TYPE ST_States :
STRUCT
	ManualModeIsActive:				BOOL;(*手动模式*)
	AutoModeIsActive:				BOOL;(*自动模式*)
	MachineRunInCycle:				BOOL;(*自动运行中*)
	GoPauseState:					BOOL;(*请求暂停记忆*)
	AutoStoping:					BOOL;(*自动停机中*)
	ResetAlarm:						BOOL;(*报警复位*)
	GoHome:							BOOL;(*请求找原点*)


	(*电机*)
	HomeDone:						BOOL;(*原点完成*)
	Motor_PowerOn:				BOOL;(*上电完成*)
	Motor_HomeDone:				BOOL;(*原点完成*)
	Motor_SwError:				BOOL;(*电机NC软件出错*)
	Motor_SwErrId:				UDINT;
	Motor_Limit:				BOOL;(*电机限位*)
	Motor_HwError:				BOOL;(*电机硬件出错*)

	Hmi_btHome:						BOOL;(*画面按钮*)(*回原点*)
	Hmi_btAutoRun:					BOOL;(*画面按钮*)(*开始*)
	Hmi_btAutoStop:					BOOL;(*画面按钮*)(*停止*)
	Hmi_btPause:					BOOL;(*画面按钮*)(*暂停*)


	(*状态*)
	ConvCanRun:						BOOL:=TRUE;(*传送带启动允许*)

	ActBoxId:						INT;(*当前进箱子的ID号*)


END_STRUCT
END_TYPE
